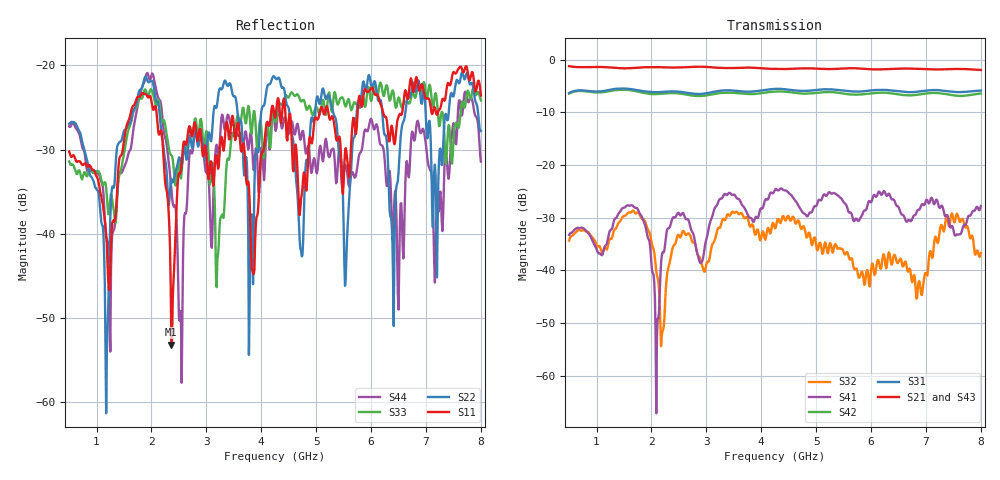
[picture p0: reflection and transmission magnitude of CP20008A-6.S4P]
!Agilent Technologies,E5071C,MY46316741,A.11.02
!Date: Fri Jun 03 17:01:18 2016
!Data & Calibration Information:
!Freq	S11:SOLT4(ON)	S12:SOLT4(ON)	S13:SOLT4(ON)	S14:SOLT4(ON)
!	S21:SOLT4(ON)	S22:SOLT4(ON)	S23:SOLT4(ON)	S24:SOLT4(ON)
!	S31:SOLT4(ON)	S32:SOLT4(ON)	S33:SOLT4(ON)	S34:SOLT4(ON)
!	S41:SOLT4(ON)	S42:SOLT4(ON)	S43:SOLT4(ON)	S44:SOLT4(ON)
!PortZ  Port1:50+j0  Port2:50+j0  Port3:50+j0  Port4:50+j0
!Above PortZ is port z conversion or system Z0 setting when saving the data.
!When reading, reference impedance value at option line is always used.
# Hz S dB R 50
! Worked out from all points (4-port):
!   601 points, 500 MHz to 8 GHz, reference 50 ohm
!   strongest paths, dB at 500 MHz, 2.375 GHz, 4.25 GHz, 6.125 GHz, 8 GHz:
!     S21: -1.2, -1.5, -1.8, -1.9, -2.0
!     S43: -1.3, -1.6, -1.9, -1.9, -2.0
!     S31: -6.3, -6.0, -5.5, -5.8, -5.9
!     S42: -6.4, -6.3, -6.1, -6.3, -6.4
!     S41: -33.3, -30.3, -24.7, -25.4, -27.8
!     S32: -34.4, -36.2, -32.0, -38.0, -36.7
!   lowest |S11| = -53.2 dB at 2.362 GHz (marker M1), VSWR 1.00, Z = 50.1 - j0.163 ohm
!   |S11| at or under -10 dB: start of sweep to end of sweep
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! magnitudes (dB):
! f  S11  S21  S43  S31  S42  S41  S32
! 500 MHz  -30.2  -1.2  -1.3  -6.3  -6.4  -33.3  -34.4
! 1.188 GHz  -41.3  -1.4  -1.5  -5.8  -6.1  -35.0  -36.1
! 1.875 GHz  -23.4  -1.4  -1.5  -6.0  -6.3  -31.2  -30.6
! 2.1 GHz  -26.1  -1.4  -1.5  -6.2  -6.5  -52.6  -41.0
! 2.362 GHz  -53.2  -1.5  -1.6  -6.0  -6.3  -30.8  -36.9
! 2.7 GHz  -27.3  -1.4  -1.5  -6.4  -6.7  -31.4  -33.3
! 8 GHz  -23.6  -2.0  -2.0  -5.9  -6.4  -27.8  -36.7
